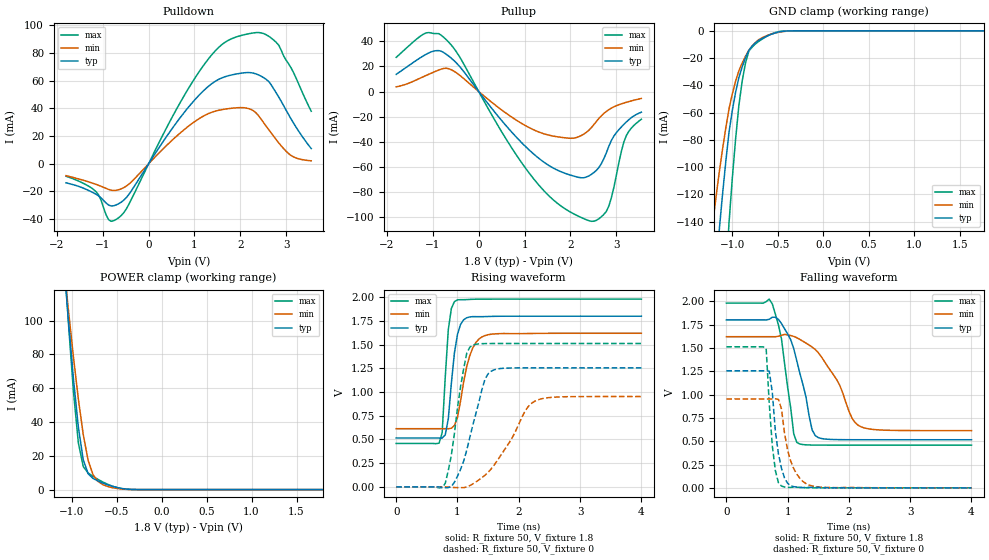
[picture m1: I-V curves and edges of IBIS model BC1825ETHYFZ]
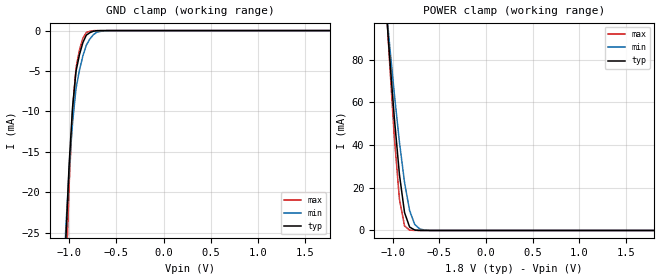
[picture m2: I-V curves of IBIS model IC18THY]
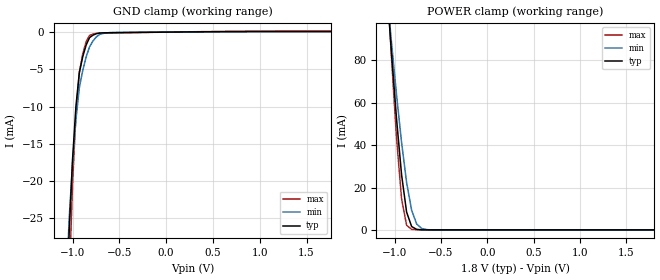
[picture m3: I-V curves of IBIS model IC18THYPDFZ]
|Texas Instruments Incorporated
[IBIS ver]   4.2
[File name]   tlk10232_noserial.ibs
[File Rev]   1.0
[Date]   Apr 26, 2013
[Source]   Texas Instruments Incorporated
[Notes]   The following is the IBIS model for the TLK10232
--Rev. 1.0:  Initial release
- IC18THYPDFZ's POWER/GND Clamp value never becomming zero reflects the behavior
  based on circuit simulation results.
- Combined Pullup/pulldown for BC1825ETHYFZ data is non-monotonic due to
  the behavior based on simulations.
[Disclaimer]
 This product is designed as an aid for customers of Texas Instruments.
 No warranties, either expressed or implied, with respect to this third
 party software (if any) or with respect to its fitness for any
 particular purpose is claimed by Texas Instruments or the author. The
 software (if any) is provided solely on an "as is" basis. The entire
 risk as to its quality and performance is with the customer
[Copyright] (C) Copyright 2013 Texas Instruments, Inc.
   All rights reserved.
|   Component tlk10232
[Component]   TLK10232
[Manufacturer]  TI
[Package]
| variable   typ   min   max
R_pkg   0.265   0.265   0.265
L_pkg   2.009n   2.009n   2.009n
C_pkg   1.172p   1.172p   1.172p
[Pin]   signal_name   model_name   R_pin   L_pin   C_pin
|  A1   INA1P   Not modeled
   A2   VSS   GND
|  A3   INA0N   Not modeled
|  A4   INA0P   Not modeled
   A5   VSS   GND
|  A6   OUTA0P   Not modeled
|  A7   OUTA0N   Not modeled
   A8   PDTRXA_N   IC18THY   0.320   2.303n   1.374p
   A9   CLKOUTBP   OCML11G   0.438   2.670n   1.108p
  A10   CLKOUTBN   OCML11G   0.440   2.828n   1.111p
  A11   VSS   GND
| A12   HSRXAN   Not modeled
|  B1   INA1N   Not modeled
|  B2   INA2P   Not modeled
   B3   VSS   GND
   B4   VSS   GND
|  B5   OUTA1P   Not modeled
|  B6   OUTA1N   Not modeled
   B7   VSS   GND
   B8   TMS   IC18THYPUFZ   0.259   2.073n   1.315p
   B9   PRBSEN   IC18THY   0.319   2.303n   1.355p
  B10   LS_OK_IN_A   IC18THY   0.357   2.574n   1.475p
  B11   VSS   GND
| B12   HSRXAP   Not modeled
   C1   VSS   GND
|  C2   INA2N   Not modeled
   C3   VDDRA_LS   POWER
|  C4   OUTA2P   Not modeled
|  C5   OUTA2N   Not modeled
   C6   VSS   GND
   C7   VDDO0   POWER
   C8   TDI   IC18THYPUFZ   0.251   2.115n   1.199p
   C9   CLKOUTAP   OCML11G   0.315   2.127n   0.904p
  C10   CLKOUTAN   OCML11G   0.317   2.140n   0.895p
| C11   AMUXA   Not modeled
  C12   VSS   GND
|  D1   INA3P   Not modeled
   D2   VDDA_LS   POWER
   D3   VSS   GND
|  D4   AMUXB   Not modeled
   D5   VSS   GND
   D6   TDO   OC1850BTFZ   0.085   1.257n   0.929p
   D7   VPP   POWER
   D8   TCK   IC18THY   0.146   1.464n   1.102p
   D9   LS_OK_OUT_A   OC1840DTFZ   0.222   1.760n   1.129p
  D10   VSS   GND
  D11   VSS   GND
| D12   HSTXAP   Not modeled
|  E1   INA3N   Not modeled
   E2   VSS   GND
|  E3   OUTA3N   Not modeled
   E4   VSS   GND
   E5   TRST_N   IC18THYPDFZ   0.142   1.344n   1.103p
   E6   VDDD   POWER
   E7   DVDD   POWER
   E8   VDDD   POWER
   E9   LOSA   OC1840DTFZ   0.171   1.512n   1.256p
  E10   PRTAD0   IC18THY   0.377   2.563n   1.434p
  E11   VDDRA_HS   POWER
| E12   HSTXAN   Not modeled
   F1   VSS   GND
   F2   VDDA_LS   POWER
|  F3   OUTA3P   Not modeled
   F4   VDDT_LS   POWER
   F5   VSS   GND
   F6   VDDD   POWER
   F7   DVDD   POWER
   F8   VSS   GND
   F9   VDDT_HS   POWER
  F10   VSS   GND
  F11   VDDA_HS   POWER
  F12   VSS   GND
   G1   VSS   GND
   G2   VDDA_LS   POWER
   G3   VSS   GND
   G4   VDDT_LS   POWER
   G5   VSS   GND
   G6   DVDD   POWER
   G7   VSS   GND
   G8   DVDD   POWER
   G9   PRTAD1   IC18THY   0.271   2.218n   1.255p
  G10   VDDA_HS   POWER
  G11   VSS   GND
| G12   HSRXBN   Not modeled
|  H1   INB0P   Not modeled
   H2   VSS   GND
|  H3   OUTB0N   Not modeled
   H4   VSS   GND
   H5   RESET_N   IC18THY   0.057   1.005n   0.864p
   H6   VDDD   POWER
   H7   DVDD   POWER
   H8   VDDD   POWER
   H9   LS_OK_OUT_B   OC1840DTFZ   0.145   1.463n   1.079p
  H10   MODE_SEL   IC18THY   0.291   2.227n   1.302p
  H11   VSS   GND
| H12   HSRXBP   Not modeled
|  J1   INB0N   Not modeled
   J2   VDDA_LS   POWER
|  J3   OUTB0P   Not modeled
   J4   PDTRXB_N   IC18THY   0.130   1.317n   0.930p
   J5   VSS   GND
   J6   PRTAD3   IC18THY   0.064   0.972n   0.936p
   J7   MDIO   BC1825ETHYFZ   0.110   1.461n   1.000p
   J8   MDC   IC18THY   0.131   1.370n   1.053p
   J9   PRBS_PASS   OC1840DTFZ   0.183   1.637n   1.123p
  J10   GPI0   IC18THY   0.265   2.118n   1.286p
  J11   VDDRB_HS   POWER
  J12   VSS   GND
   K1   VSS   GND
|  K2   INB1P   Not modeled
   K3   VDDRB_LS   POWER
|  K4   OUTB1N   Not modeled
|  K5   OUTB1P   Not modeled
   K6   VSS   GND
   K7   VDDO1   POWER
   K8   LOSB   OC1840DTFZ   0.205   1.920n   1.163p
   K9   REFCLK1P   ICLKRX18G   0.313   2.156n   0.909p
  K10   REFCLK1N   ICLKRX18G   0.315   2.161n   0.913p
  K11   VSS   GND
| K12   HSTXBP   Not modeled
|  L1   INB2P   Not modeled
|  L2   INB1N   Not modeled
   L3   VSS   GND
   L4   VSS   GND
|  L5   OUTB2N   Not modeled
|  L6   OUTB2P   Not modeled
   L7   VSS   GND
   L8   LS_OK_IN_B   IC18THY   0.297   2.183n   1.382p
   L9   PRTAD2   IC18THY   0.283   1.981n   1.339p
  L10   TESTEN   IC18THY   0.345   2.243n   1.448p
  L11   VSS   GND
| L12   HSTXBN   Not modeled
|  M1   INB2N   Not modeled
   M2   VSS   GND
|  M3   INB3P   Not modeled
|  M4   INB3N   Not modeled
   M5   VSS   GND
|  M6   OUTB3N   Not modeled
|  M7   OUTB3P   Not modeled
   M8   PRTAD4   IC18THY   0.369   2.415n   1.483p
   M9   ST   IC18THY   0.384   2.667n   1.507p
  M10   REFCLK0P   ICLKRX18G   0.476   2.906n   1.190p
  M11   REFCLK0N   ICLKRX18G   0.478   2.851n   1.184p
  M12   VSS   GND
[Diff Pin]   inv_pin  vdiff   tdelay_typ  tdelay_min  tdelay_max
M10   M11   200mV   NA   NA   NA
K9   K10   200mV   NA   NA   NA
C9   C10   200mV   NA   NA   NA
A9   A10   200mV   NA   NA   NA
| Models and submodels in the file (8): BC1825ETHYFZ (I/O), IC18THY (Input), IC18THYPDFZ (Input), IC18THYPUFZ (Input), ICLKRX18G (Input), OC1840DTFZ (3-state), OC1850BTFZ (3-state), OCML11G (Output)
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[Model]   BC1825ETHYFZ
Model_type   I/O
Polarity   Non-Inverting
Enable   Active-Low
Vinl =  0.63
Vinh =  1.17
Cref =  15.0000pF
Rref =  100.0000M
Vref =  0V
Vmeas =  0.9
C_comp   1.756427p   1.323266p   2.339455p
[Model Spec]
Vinl   0.63   0.567   0.693
Vinh   1.17   1.053   1.287
[Temperature Range]   25   125   -40
[Voltage Range]   1.8   1.62   1.98
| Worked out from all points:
|   slope of the pulldown table from 0 to 0.27 V, typ, clamps not added: 19.6 ohm
|   slope of the pullup table from 0 to 0.27 V, typ, clamps not added: 21.2 ohm
|   GND clamp passes 1 mA (typ) near -0.50 V on its own axis
|   POWER clamp passes 1 mA (typ) near -0.48 V on its own axis
|   rising waveform, R_fixture 50, V_fixture 1.8: 20-80 % time 126ps typ, 198ps min, 87.5ps max; typ from 0.516 V to 1.8 V
|   rising waveform, R_fixture 50, V_fixture 0: 20-80 % time 302ps typ, 522ps min, 201ps max; typ from 0 V to 1.25 V
|   falling waveform, R_fixture 50, V_fixture 1.8: 20-80 % time 277ps typ, 470ps min, 194ps max; typ from 1.8 V to 0.516 V
|   falling waveform, R_fixture 50, V_fixture 0: 20-80 % time 134ps typ, 197ps min, 104ps max; typ from 1.25 V to 0 V
[POWER_clamp]
-1.8V     671.8mA    545.1mA    808.2mA
-1.073V   123.7mA    124.6mA    127.1mA
-1.055V   111.5mA    115mA      112.4mA
-981.8mV  65.6mA     78.46mA    58.15mA
-927.3mV  37.01mA    53.65mA    27.72mA
-872.7mV  17.65mA    32.56mA    13.64mA
-818.2mV  9.375mA    17.27mA    9.824mA
-763.6mV  6.606mA    8.774mA    7.806mA
-654.5mV  3.864mA    2.942mA    4.49mA
-490.9mV  1.152mA    622.6uA    1.11mA
-327.3mV  85.89uA    40.76uA    54.47uA
1.8V      224.8nA    189.7nA    319.8nA
[Pulldown]
-1.8V     -13.79mA   -8.604mA   -9.047mA
-1.145V   -22.07mA   -14.92mA   -20.24mA
-872.7mV  -29.86mA   -18.56mA   -40.41mA
-654.5mV  -28.9mA    -18.77mA   -39.05mA
-436.4mV  -22.41mA   -14.91mA   -29.64mA
1.091V    49.25mA    32.39mA    66.03mA
1.582V    61.86mA    39.02mA    85.71mA
2.018V    65.47mA    40.6mA     92.73mA
2.345V    64.89mA    36.67mA    94.82mA
2.782V    51.24mA    17.42mA    87.77mA
3.109V    32.2mA     5.915mA    69.14mA
3.545V    10.99mA    2.102mA    37.97mA
[Pullup]
-1.8V     13.68mA    3.76mA     27.17mA
-1.145V   29.68mA    12.85mA    46.61mA
-763.6mV  30.98mA    18.39mA    43.09mA
-436.4mV  20.7mA     13.56mA    28.7mA
545.5mV   -25mA      -15.84mA   -34.72mA
1.2V      -49.7mA    -30.43mA   -69.45mA
2.018V    -66.57mA   -37.11mA   -96.11mA
2.4V      -67.01mA   -30.75mA   -102.6mA
2.782V    -48.63mA   -15.78mA   -95.19mA
2.891V    -38.89mA   -13.16mA   -84.37mA
3.164V    -26.08mA   -9.131mA   -40.05mA
3.545V    -16.39mA   -5.461mA   -21.97mA
[GND_clamp]
-1.8V     -733.8mA   -497.1mA   -1.291A
-1.218V   -206.8mA   -143.2mA   -384.4mA
-1.145V   -148mA     -104.9mA   -278.9mA
-1.109V   -121.5mA   -87.8mA    -229.9mA
-1.036V   -74.74mA   -57.48mA   -141.5mA
-963.6mV  -45.13mA   -37mA      -79.59mA
-927.3mV  -34.3mA    -29.23mA   -54.66mA
-890.9mV  -26.43mA   -23.61mA   -36.81mA
-818.2mV  -14.35mA   -14.32mA   -14.96mA
-709.1mV  -6.982mA   -6.478mA   -7.736mA
-418.2mV  -220.1uA   -368.1uA   -103.1uA
1.764V    204.4nA    959.6nA    204.4nA
[Ramp]
dV/dt_f  0.7911936/0.2872552n  0.6188735/0.488238n   0.9397716/0.2004116n
dV/dt_r  0.7583382/0.3036187n  0.5768991/0.5283491n  0.9134414/0.2030853n
R_load = 50
[Rising Waveform]
R_fixture = 50
V_fixture = 1.8
V_fixture_min = 1.62
V_fixture_max = 1.98
0s        515.6mV    613.4mV    457.9mV
700ps     515.4mV    613.4mV    461.2mV
750ps     515.1mV    613.5mV    571.5mV
800ps     548.3mV    613.7mV    1.155V
850ps     717.4mV    612.7mV    1.659V
900ps     1.093V     618.5mV    1.881V
1ns       1.609V     733.8mV    1.973V
1.2ns     1.792V     1.383V     1.977V
1.4ns     1.795V     1.582V     1.98V
4ns       1.8V       1.62V      1.98V
[Rising Waveform]
R_fixture = 50
V_fixture = 0
V_fixture_min = 0
V_fixture_max = 0
0s        770.2nV    748.4nV    867.8nV
800ps     -9.101mV   337.4uV    36.46mV
950ps     49.28mV    -7.17mV    563.1mV
1.05ns    184.9mV    -8.299mV   1.058V
1.15ns    385.1mV    -1.425mV   1.407V
1.25ns    651.6mV    31.2mV     1.495V
1.4ns     1.03V      97.98mV    1.51V
1.5ns     1.193V     153.4mV    1.512V
2.25ns    1.255V     899.5mV    1.512V
4ns       1.255V     952.8mV    1.512V
[Falling Waveform]
R_fixture = 50
V_fixture = 1.8
V_fixture_min = 1.62
V_fixture_max = 1.98
0s        1.8V       1.62V      1.98V
750ps     1.829V     1.62V      1.972V
900ps     1.761V     1.635V     1.596V
1.1ns     1.492V     1.623V     577.9mV
1.15ns    1.36V      1.609V     486.6mV
1.4ns     620.2mV    1.509V     458.9mV
1.5ns     538.6mV    1.449V     458.2mV
2.05ns    515.9mV    747.8mV    457.9mV
2.2ns     515.7mV    653.5mV    457.9mV
4ns       515.6mV    613.4mV    457.9mV
[Falling Waveform]
R_fixture = 50
V_fixture = 0
V_fixture_min = 0
V_fixture_max = 0
0s        1.255V     952.8mV    1.512V
650ps     1.255V     952.8mV    1.493V
700ps     1.252V     952.8mV    905.1mV
750ps     1.025V     952.7mV    450.9mV
800ps     607.6mV    954.1mV    185.8mV
900ps     209.2mV    844.8mV    18.9mV
950ps     105.4mV    583.9mV    9.035mV
1.05ns    23.66mV    287.8mV    4.752mV
1.35ns    5.405mV    30.23mV    1.017mV
4ns       770.2nV    1.66uV     867.8nV
[Model]   IC18THY
Model_type   Input
Polarity   Non-Inverting
Vinl =  0.63
Vinh =  1.17
C_comp   0.6387869p   0.5480567p   0.7549689p
[Model Spec]
Vinl   0.63   0.5985   0.6615
Vinh   1.17   1.1115   1.2285
[Temperature Range]   25   125   -40
[Voltage Range]   1.8   1.71   1.89
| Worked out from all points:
|   GND clamp passes 1 mA (typ) near -0.84 V on its own axis
|   POWER clamp passes 1 mA (typ) near -0.79 V on its own axis
[POWER_clamp]
-1.8V     607mA      492.8mA    733.5mA
-1.055V   94.75mA    97.21mA    95.13mA
-1.036V   83.56mA    88.51mA    81.22mA
-981.8mV  52.51mA    63.81mA    43.47mA
-927.3mV  26.09mA    41.33mA    14.63mA
-872.7mV  8.397mA    22.47mA    2.133mA
-818.2mV  1.587mA    9.312mA    180.8uA
-763.6mV  228.2uA    2.824mA    13.3uA
-709.1mV  29.94uA    699uA      954.2nA
-654.5mV  3.826uA    158.9uA    68.5nA
1.8V      3.537pA    1.47pA     16.11pA
[GND_clamp]
-1.8V     -539.1mA   -380.2mA   -748.9mA
-1.036V   -26.23mA   -24.68mA   -32.15mA
-1V       -16.52mA   -17.21mA   -19.02mA
-963.6mV  -9.451mA   -11.37mA   -9.842mA
-927.3mV  -5.032mA   -7.151mA   -4.619mA
-890.9mV  -2.977mA   -4.906mA   -2.412mA
-854.5mV  -1.487mA   -3.125mA   -949uA
-818.2mV  -563.1uA   -1.808mA   -231uA
-781.8mV  -269.9uA   -1.064mA   -91.3uA
-709.1mV  -19.12uA   -213.6uA   -1.453uA
-600mV    -278.7nA   -13.18uA   -6.862nA
1.764V    3.096pA    9.108pA    10.16pA
[Model]   IC18THYPDFZ
Model_type   Input
Polarity   Non-Inverting
Vinl =  0.63
Vinh =  1.17
C_comp   0.7118224p   0.6228336p   0.8322228p
[Model Spec]
Vinl   0.63   0.5985   0.6615
Vinh   1.17   1.1115   1.2285
[Temperature Range]   25   125   -40
[Voltage Range]   1.8   1.71   1.89
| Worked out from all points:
|   GND clamp passes 1 mA (typ) near -0.83 V on its own axis
|   POWER clamp passes 1 mA (typ) near -0.79 V on its own axis
[POWER_clamp]
-1.8V     607.1mA    492.9mA    733.7mA
-1.055V   94.83mA    97.26mA    95.27mA
-1.036V   83.65mA    88.56mA    81.36mA
-981.8mV  52.59mA    63.87mA    43.61mA
-927.3mV  26.18mA    41.38mA    14.77mA
-872.7mV  8.488mA    22.52mA    2.281mA
-818.2mV  1.679mA    9.367mA    329.5uA
-763.6mV  320.4uA    2.879mA    161.9uA
-709.1mV  122uA      754.7uA    149.4uA
-654.5mV  95.78uA    214.5uA    148.3uA
1.8V      90.13uA    54.48uA    145.3uA
[GND_clamp]
-1.8V     -542mA     -381.8mA   -757.7mA
-1.073V   -42.86mA   -36.02mA   -57.35mA
-1.036V   -26.92mA   -25.12mA   -33.88mA
-1V       -17.11mA   -17.6mA    -20.43mA
-963.6mV  -9.945mA   -11.71mA   -10.93mA
-927.3mV  -5.429mA   -7.442mA   -5.388mA
-890.9mV  -3.287mA   -5.15mA    -2.922mA
-854.5mV  -1.723mA   -3.324mA   -1.27mA
-818.2mV  -734.7uA   -1.966mA   -430.8uA
-709.1mV  -120uA     -294.3uA   -144.9uA
-600mV    -81.62uA   -67.48uA   -118.2uA
1.764V    90uA       54.59uA    144.6uA
